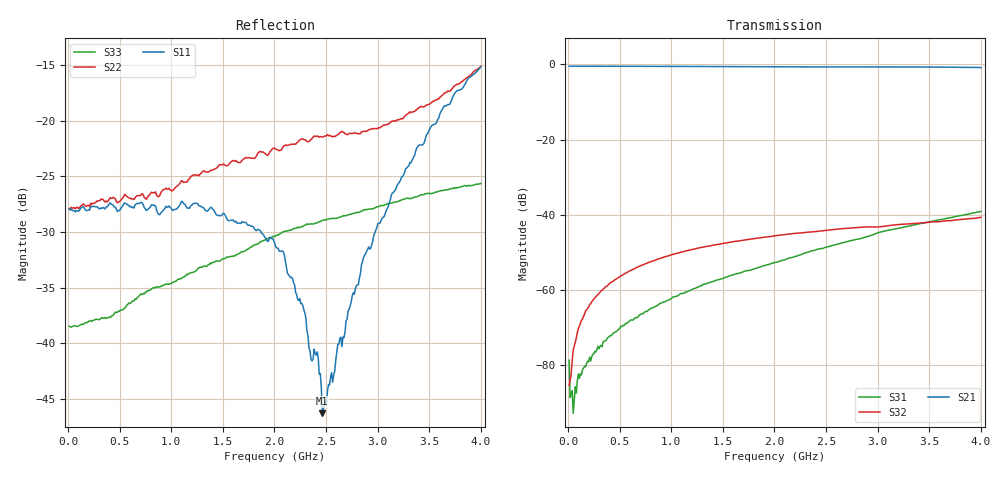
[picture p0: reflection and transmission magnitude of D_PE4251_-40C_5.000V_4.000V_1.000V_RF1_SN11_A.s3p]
! Device ID: PE4251_SoldCshunt_081809
! Dir: c:\Test Bench Repositories\Bench_Software_CVI_Version_8\trunk\PSC 4Port_VNA Bench\datalog\4250\TEST\PE4251_SoldCshunt_081809\-40C\5p000000\RF1
! Serial: 11
! Insertion: A
! Temp: -40C
! VDD: 5.000
! Control_Hi: 80.000
! Control_Lo: 20.000
! Logic State: RF1
! Port 1: RFC
! Port 2: RF1
! Port 3: RF2
! V1 = 1.00
! V2 = 4.00
! V3 = 1.00
! IDD: 5.914020e-05
! FILE NAME
! DATE 08/18/09  20:10
! CORRECTED  DATA
#  Hz  S  RI  R  50.00
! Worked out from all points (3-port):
!   401 points, 10 MHz to 4 GHz, reference 50 ohm
!   strongest paths, dB at 10 MHz, 1.008 GHz, 2.005 GHz, 3.002 GHz, 4 GHz:
!     S21: -0.5, -0.5, -0.6, -0.7, -0.9
!     S32: -85.5, -50.6, -45.7, -43.3, -40.7
!     S31: -78.7, -62.2, -52.7, -44.8, -39.2
!   lowest |S11| = -46.3 dB at 2.464 GHz (marker M1), VSWR 1.01, Z = 50.2 - j0.457 ohm
!   |S11| at or under -10 dB: start of sweep to end of sweep
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1e7  0.0402 4.48e-05  0.9443 -0.00289  4.97e-05 -0.000117
     0.945 -0.00406  0.0403 0.000225  -2.46e-06 0.00015
     0.000115 -1.51e-05  2.4e-05 -4.75e-05  0.0119 -0.000406
3.9925e7  0.0395 -0.000193  0.9456 -0.0155  1.7e-05 -4.22e-05
          0.946 -0.0155  0.0404 -0.000133  3.08e-05 0.000119
          8.81e-06 -4.44e-05  3.52e-05 0.000109  0.0119 0.000156
1.8955e8  0.0395 0.000321  0.9428 -0.0647  -1.06e-05 -9.89e-05
          0.9426 -0.0645  0.0416 -0.000126  5.24e-05 0.000566
          -1.14e-05 -0.000111  4.64e-05 0.000566  0.0123 0.00162
4.98775e8  0.0394 -0.00251  0.928 -0.1659  -0.000157 -0.000255
           0.9286 -0.1651  0.0433 -0.00208  0.000143 0.00149
           -0.000159 -0.000258  0.000151 0.00149  0.0134 0.00383
1.10725e9  0.0411 -0.0141  0.8699 -0.3544  -0.000782 -0.000431
           0.8705 -0.3541  0.0516 -0.0148  0.000583 0.00313
           -0.000778 -0.000437  0.000574 0.00312  0.0164 0.0109
2.005e9  0.026 -0.0102  0.7218 -0.5846  -0.00226 -0.00045
         0.7219 -0.5843  0.0662 -0.0355  0.00121 0.00506
         -0.00227 -0.000455  0.00122 0.00507  0.0185 0.0238
2.2843e9  0.0109 -0.00903  0.6662 -0.6444  -0.003 -0.00054
          0.665 -0.6452  0.0645 -0.0511  0.00139 0.00558
          -0.003 -0.000554  0.00138 0.0056  0.017 0.0291
2.46385e9  0.00163 -0.00456  0.6291 -0.6796  -0.0035 -0.000495
           0.6277 -0.6796  0.0613 -0.0579  0.00139 0.00591
           -0.00352 -0.000497  0.00139 0.00594  0.0155 0.032
3.14215e9  -0.0365 -0.0302  0.4633 -0.8007  -0.00634 -1.08e-05
           0.4648 -0.8003  0.0221 -0.097  0.00118 0.00713
           -0.00634 -4.19e-05  0.00119 0.00714  0.00699 0.0421
4e9  -0.1568 -0.0773  0.1828 -0.8903  -0.0108 0.00215
     0.1818 -0.8867  -0.1202 -0.1284  7.01e-05 0.00918
     -0.0108 0.0021  4.57e-05 0.0092  -0.0133 0.0505
